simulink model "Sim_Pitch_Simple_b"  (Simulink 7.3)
settings: Solver=ode23s  StartTime=0.0  StopTime=20  RelTol=1e-3
InitFcn:
  | init
StartFcn:
  | init
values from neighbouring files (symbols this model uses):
  d2r = pi/180    (= 0.0174532925199)    [init.m]    (also in robust.m)
  r2d = 180/pi    (= 57.2957795131)    [init.m]    (also in robust.m)
undefined symbols (not defined in the file or in its folder): Aps, Bps, Cps, Dps, Kmix, Kq

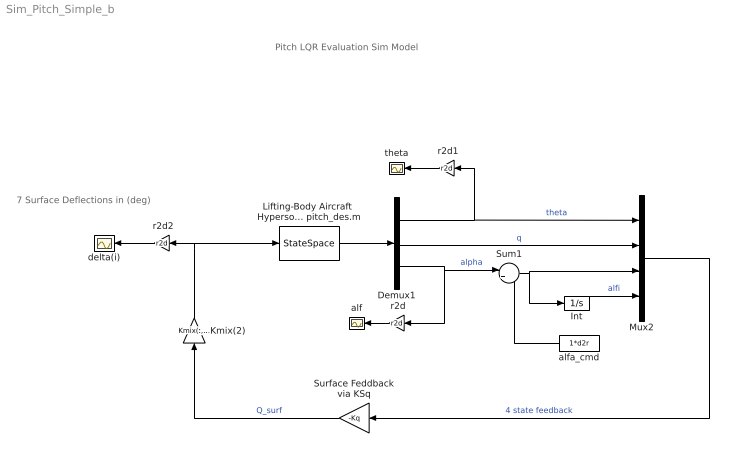
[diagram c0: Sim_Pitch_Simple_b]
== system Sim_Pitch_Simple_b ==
  note: 7 Surface Deflections in (deg)
  note: Pitch LQR Evaluation Sim Model
  " r2d" : Gain  Gain=r2d  ParameterDataType=sfix(16)  ParameterScaling=2^0  OutDataType=sfix(16)  OutScaling=2^0
  " r2d1" : Gain  Gain=r2d  ParameterDataType=sfix(16)  ParameterScaling=2^0  OutDataType=sfix(16)  OutScaling=2^0
  " r2d2" : Gain  Gain=r2d  ParameterDataType=sfix(16)  ParameterScaling=2^0  OutDataType=sfix(16)  OutScaling=2^0
  Demux1 : Demux  Outputs=3
  Int : Integrator
  Kmix(2) : Gain  Gain=Kmix(:,2)  Multiplication=Matrix(K*u)  ParameterDataType=sfix(16)  ParameterScaling=2^0  OutDataType=sfix(16)  OutScaling=2^0
  Lifting-Body Aircraft  Hypersonic Pitch  Design Model from file pitch_des.m : StateSpace  A=Aps  B=Bps  C=Cps  D=Dps
  Mux2 : Mux
  Sum1 : Sum  Inputs=|+-  OutDataType=sfix(16)  OutScaling=2^0
  Surface Feddback via KSq : Gain  Gain=-Kq  Multiplication=Matrix(K*u)  ParameterDataType=sfix(16)  ParameterScaling=2^0  OutDataType=sfix(16)  OutScaling=2^0
  alf : Scope
  alfa_cmd : Constant  Value=1*d2r  OutDataType=sfix(16)  OutScaling=2^0
  delta(i) : Scope
  theta : Scope
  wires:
  Demux1/2 -> Mux2/2  "q"
  Mux2/1 -> Surface Feddback via KSq/1  "4 state feedback"
  Surface Feddback via KSq/1 -> Kmix(2)/1  "Q_surf"
  " r2d"/1 -> alf/1
  Lifting-Body Aircraft  Hypersonic Pitch  Design Model from file pitch_des.m/1 -> Demux1/1
  Demux1/3 -> " r2d"/1, Sum1/1  "alpha"
  Demux1/1 -> " r2d1"/1, Mux2/1  "theta"
  " r2d1"/1 -> theta/1
  Kmix(2)/1 -> Lifting-Body Aircraft  Hypersonic Pitch  Design Model from file pitch_des.m/1, " r2d2"/1
  " r2d2"/1 -> delta(i)/1
  Int/1 -> Mux2/4  "alfi"
  Sum1/1 -> Mux2/3, Int/1
  alfa_cmd/1 -> Sum1/2
